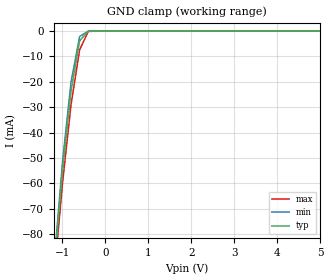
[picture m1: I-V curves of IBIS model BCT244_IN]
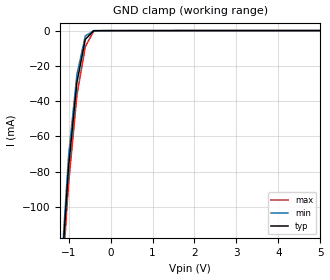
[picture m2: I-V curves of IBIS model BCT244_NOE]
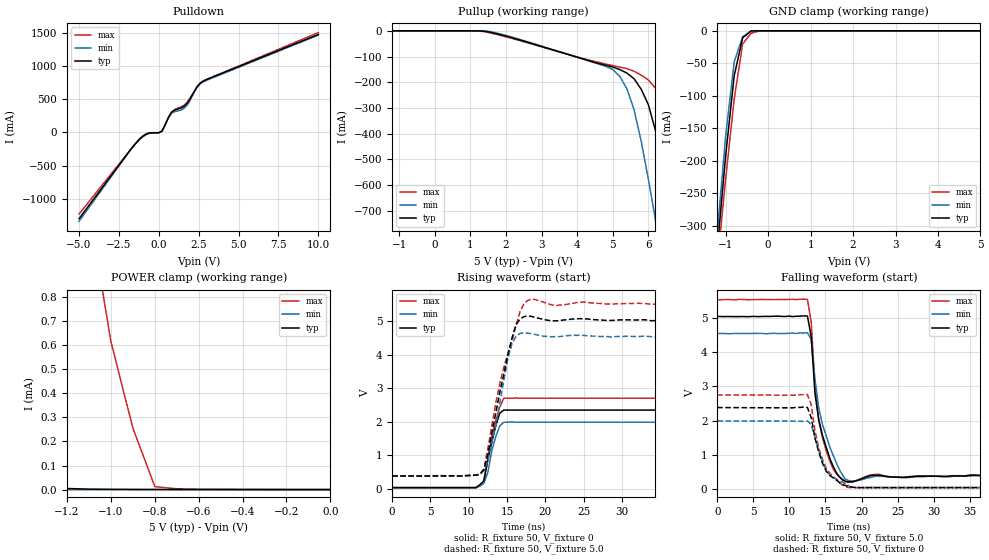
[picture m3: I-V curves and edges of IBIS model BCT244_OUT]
|   TEXAS INSTRUMENTS INCORPORATED
|   Standard Linear and Logic
|   IBIS Model of SN74BCT244
|   OCTAL BUFFERS / DRIVERS WITH 3-STATE OUTPUTS
|   SOIC 20-pin (DW), SOP 20-pin (NS), SSOP 20-pin (DB), PDIP 20-pin (N)
[IBIS Ver]   3.2
[Comment Char]  |_char
[File Name]   sn74bct244.ibs
[File Rev]   4.2 | b_die
[Date]   Oct. 06, 2004
[Source]   File originated at Texas Instruments, Inc.
[Notes]   The following is a sample IBIS file for the BCT244
   - FILE REV HISTORY
   - 4.2 Re-Release IBIS file on 10/08/04
   - All test data contained in this file are derived from
   actual measurements.
   - The measurement used NS package.
   - We have data across voltage and temperature, but not
   across process.
   - As there is no power clamp diode we removed the Pwr Clamp
   table data for IN and NOE.
|   - File created by Nobuhisa Ohtsubo, SLL Product Engineering.
[Disclaimer] Property of Texas Instruments Incorporated.  Unauthorized
   reproduction and/or distribution is strictly prohibited.
   This product is protected under copyright law.
   Created 2000, (C) Copyright 2000, Texas Instruments Inc.,
   All Rights Reserved.
   UNLESS THERE IS A SIGNED, WRITTEN AGREEMENT TO THE
   CONTRARY, TEXAS INSTRUMENTS () IS PROVIDING THE IBIS
   MODELS  AND WITHOUT ANY WARRANTY, EXPRESSED OR
   IMPLIED.  TI assumes no liability for:
   1) the accuracy of the IBIS models provided to your
   company;
   2) the proper functioning of these IBIS Models in your
   design or for any resulting applications; or
   3) infringement of patents, copyrights or intellectual
   property rights resulting from your use of these IBIS
   models.
   TI provides IBIS Models as a service to our customers.
   You and your company shall not distribute, sell or give
   these models to anyone else without prior written
   permission from TI.
   TI reserves the right to make changes to our products or
   to discontinue any semiconductor product or service
   without notice, and advises our customers to obtain the
   latest version of relevant information to verify, before
   placing orders, that the information being relied on is
   current.
   Please be aware that your receipt and use of the IBIS
   information provided shall serve as acceptance of these
   terms and conditions.  If you do not accept these terms,
   you should return or destroy the IBIS models and any
   other accompanying information immediately.
|   Component BCT244_DW
[Component]   BCT244_DW
[Manufacturer]  Texas Instruments, Inc.
[Package]
|   typ   min   max
R_pkg   0.038   0.033   0.045
L_pkg   5.012nH   4.110nH   6.349nH
C_pkg   0.717pF   0.530pF   0.868pF
[Pin]   signal_name   model_name   R_pin   L_pin   C_pin
1   1NOE   BCT244_NOE   0.058   5.115nH   0.725pF
2   1A1   BCT244_IN   0.053   4.591nH   0.724pF
3   2Y4   BCT244_OUT   0.049   3.754nH   0.572pF
4   1A2   BCT244_IN   0.029   2.549nH   0.388pF
5   2Y3   BCT244_OUT   0.031   2.317nH   0.316pF
6   1A3   BCT244_IN   0.031   2.317nH   0.316pF
7   2Y2   BCT244_OUT   0.029   2.556nH   0.399pF
8   1A4   BCT244_IN   0.049   3.754nH   0.579pF
9   2Y1   BCT244_OUT   0.053   4.591nH   0.724pF
10   GND   GND   0.058   5.115nH   0.725pF
11   2A1   BCT244_IN   0.058   5.115nH   0.725pF
12   1Y4   BCT244_OUT   0.053   4.591nH   0.724pF
13   2A2   BCT244_IN   0.049   3.754nH   0.579pF
14   1Y3   BCT244_OUT   0.029   2.557nH   0.399pF
15   2A3   BCT244_IN   0.031   2.317nH   0.316pF
16   1Y2   BCT244_OUT   0.031   2.317nH   0.316pF
17   2A4   BCT244_IN   0.029   2.557nH   0.399pF
18   1Y1   BCT244_OUT   0.049   3.754nH   0.579pF
19   2NOE   BCT244_NOE   0.053   4.591nH   0.724pF
20   VCC   POWER   0.058   5.115nH   0.725pF
|   Component BCT244_NS
[Component]   BCT244_NS
[Manufacturer]  Texas Instruments, Inc.
[Package]
|   typ   min   max
R_pkg   0.044   0.029   0.058
L_pkg   3.666nH   2.317nH   5.115nH
C_pkg   0.548pF   0.316pF   0.725pF
[Pin]   signal_name   model_name   R_pin   L_pin   C_pin
1   1NOE   BCT244_NOE   0.058   5.115nH   0.725pF
2   1A1   BCT244_IN   0.053   4.591nH   0.724pF
3   2Y4   BCT244_OUT   0.049   3.754nH   0.572pF
4   1A2   BCT244_IN   0.029   2.549nH   0.388pF
5   2Y3   BCT244_OUT   0.031   2.317nH   0.316pF
6   1A3   BCT244_IN   0.031   2.317nH   0.316pF
7   2Y2   BCT244_OUT   0.029   2.556nH   0.399pF
8   1A4   BCT244_IN   0.049   3.754nH   0.579pF
9   2Y1   BCT244_OUT   0.053   4.591nH   0.724pF
10   GND   GND   0.058   5.115nH   0.725pF
11   2A1   BCT244_IN   0.058   5.115nH   0.725pF
12   1Y4   BCT244_OUT   0.053   4.591nH   0.724pF
13   2A2   BCT244_IN   0.049   3.754nH   0.579pF
14   1Y3   BCT244_OUT   0.029   2.557nH   0.399pF
15   2A3   BCT244_IN   0.031   2.317nH   0.316pF
16   1Y2   BCT244_OUT   0.031   2.317nH   0.316pF
17   2A4   BCT244_IN   0.029   2.557nH   0.399pF
18   1Y1   BCT244_OUT   0.049   3.754nH   0.579pF
19   2NOE   BCT244_NOE   0.053   4.591nH   0.724pF
20   VCC   POWER   0.058   5.115nH   0.725pF
|   Component BCT244_DB
[Component]   BCT244_DB
[Manufacturer]  Texas Instruments, Inc.
[Package]
|   typ   min   max
R_pkg   0.040   0.035   0.051
L_pkg   3.495nH   3.035nH   4.314nH
C_pkg   0.420pF   0.346pF   0.502pF
[Pin]   signal_name   model_name   R_pin   L_pin   C_pin
1   1NOE   BCT244_NOE   0.049   4.310nH   0.502pF
2   1A1   BCT244_IN   0.048   3.903nH   0.487pF
3   2Y4   BCT244_OUT   0.035   3.189nH   0.396pF
4   1A2   BCT244_IN   0.035   3.036nH   0.347pF
5   2Y3   BCT244_OUT   0.035   3.035nH   0.367pF
6   1A3   BCT244_IN   0.035   3.035nH   0.367pF
7   2Y2   BCT244_OUT   0.035   3.036nH   0.347pF
8   1A4   BCT244_IN   0.035   3.189nH   0.397pF
9   2Y1   BCT244_OUT   0.047   3.899nH   0.488pF
10   GND   GND   0.051   4.314nH   0.500pF
11   2A1   BCT244_IN   0.051   4.314nH   0.500pF
12   1Y4   BCT244_OUT   0.047   3.899nH   0.488pF
13   2A2   BCT244_IN   0.035   3.189nH   0.397pF
14   1Y3   BCT244_OUT   0.035   3.036nH   0.346pF
15   2A3   BCT244_IN   0.035   3.035nH   0.367pF
16   1Y2   BCT244_OUT   0.035   3.035nH   0.367pF
17   2A4   BCT244_IN   0.035   3.036nH   0.346pF
18   1Y1   BCT244_OUT   0.035   3.189nH   0.397pF
19   2NOE   BCT244_NOE   0.047   3.899nH   0.488pF
20   VCC   POWER   0.051   4.314nH   0.502pF
|   Component BCT244_N
[Component]   BCT244_N
[Manufacturer]   Texas Instruments, Inc.
[Package]
|   typ   min   max
R_pkg   4.300e-02   3.800e-02   5.000e-02
L_pkg   7.384e-09   4.680e-09   1.032e-08
C_pkg   5.100e-13   2.310e-13   8.210e-13
[PIN]   signal_name   model_name   R_pin   L_pin   C_pin
1   1NOE   BCT244_NOE   4.200e-02   9.427e-09   8.100e-13
2   1A1   BCT244_IN   4.600e-02   8.544e-09   4.560e-13
3   2Y4   BCT244_OUT   4.800e-02   7.163e-09   4.350e-13
4   1A2   BCT244_IN   4.000e-02   4.825e-09   2.610e-13
5   2Y3   BCT244_OUT   4.000e-02   5.284e-09   6.480e-13
6   1A3   BCT244_IN   4.000e-02   4.686e-09   2.320e-13
7   2Y2   BCT244_OUT   4.000e-02   6.359e-09   4.890e-13
8   1A4   BCT244_IN   3.800e-02   7.982e-09   4.750e-13
9   2Y1   BCT244_OUT   4.300e-02   9.403e-09   4.750e-13
10   GND   GND   5.000e-02   1.032e-08   8.050e-13
11   2A1   BCT244_IN   5.000e-02   1.028e-08   8.100e-13
12   1Y4   BCT244_OUT   4.300e-02   9.383e-09   4.770e-13
13   2A2   BCT244_IN   3.800e-02   7.978e-09   4.760e-13
14   1Y3   BCT244_OUT   4.000e-02   6.302e-09   4.920e-13
15   2A3   BCT244_IN   4.000e-02   4.680e-09   2.310e-13
16   1Y2   BCT244_OUT   4.000e-02   5.284e-09   6.480e-13
17   2A4   BCT244_IN   4.000e-02   4.822e-09   2.610e-13
18   1Y1   BCT244_OUT   4.700e-02   7.118e-09   4.390e-13
19   2NOE   BCT244_NOE   4.600e-02   8.492e-09   4.610e-13
20   VCC   POWER   4.300e-02   9.348e-09   8.210e-13
| Models and submodels in the file (3): BCT244_IN (Input), BCT244_NOE (Input), BCT244_OUT (3-state)
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|   Model BCT244_IN
[Model]   BCT244_IN
Model_type  Input
Polarity   Inverting
Vinl = 0.8
Vinh = 2.0
| variable   typ   min   max
C_comp   1.33pf   1.00pf   1.66pf
[Temperature Range]   25   0   70
[Voltage Range]   5.0   4.5   5.5
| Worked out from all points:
|   GND clamp passes 1 mA (typ) near -0.45 V on its own axis
[GND Clamp]
|   Voltage   I(typ)   I(min)   I(max)
-5V       -1.129A    -1.189A    -1.042A
-1.2V     -95.01mA   -92.75mA   -98.11mA
-1V       -55.16mA   -51.8mA    -60.26mA
-800mV    -23.57mA   -20.06mA   -29.07mA
-600mV    -3.849mA   -2.148mA   -7.399mA
-400mV    -30.54uA   -20.12uA   -154.2uA
5V        3.151nA    4.209nA    5.215nA
|   Model BCT244_NOE
[Model]   BCT244_NOE
Model_type  Input
Polarity   Inverting
Vinl = 0.8
Vinh = 2.0
| variable   typ   min   max
C_comp   1.33pf   1.00pf   1.66pf
[Temperature Range]   25   0   70
[Voltage Range]   5.0   4.5   5.5
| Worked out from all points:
|   GND clamp passes 1 mA (typ) near -0.44 V on its own axis
[GND Clamp]
|   Voltage   I(typ)   I(min)   I(max)
-5V       -1.905A    -1.987A    -1.775A
-1.2V     -149.5mA   -144.7mA   -156.5mA
-1V       -77.36mA   -71.2mA    -87.15mA
-800mV    -29.14mA   -24.72mA   -36.51mA
-600mV    -4.94mA    -2.996mA   -9.102mA
-400mV    -73.28uA   -48.98uA   -291.7uA
5V        3.575nA    6.334nA    4.663nA
|   Model BCT244_OUT
[Model]   BCT244_OUT
Model_type  3-state
Polarity   Non-Inverting
Vmeas = 1.3v
Cref = 50pF
Rref = 500
Vref = 0
| variable   typ   min   max
C_comp   5.8pf   4.35pf   7.25pf
[Temperature Range]   25   0   70
[Voltage Range]   5.0   4.5   5.5
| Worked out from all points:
|   slope of the pulldown table from 0 to 0.75 V, typ, clamps not added: 2.58 ohm
|   slope of the pullup table from 0 to 0.75 V, typ, clamps not added: 69.6 kohm
|   GND clamp passes 1 mA (typ) near -0.41 V on its own axis
|   POWER clamp passes 1 mA (typ) near -1.49 V on its own axis
|   rising waveform, R_fixture 50, V_fixture 0: 20-80 % time 1.33ns typ, 1.2ns min, 1.48ns max; typ from 0.031 V to 2.35 V
|   falling waveform, R_fixture 50, V_fixture 5.0: 20-80 % time 1.83ns typ, 2.31ns min, 1.56ns max; typ from 5.05 V to 0.385 V
|   rising waveform, R_fixture 50, V_fixture 5.0: 20-80 % time 2.5ns typ, 2.1ns min, 3.1ns max; typ from 0.375 V to 5.05 V
|   falling waveform, R_fixture 50, V_fixture 0: 20-80 % time 1.97ns typ, 2.1ns min, 1.95ns max; typ from 2.38 V to 0.038 V
[Pulldown]
|   Voltage   I(typ)   I(min)   I(max)
-5V       -1.301A    -1.34A     -1.231A
-1.4V     -150mA     -146.8mA   -155.5mA
-800mV    -25.67mA   -22.18mA   -32.16mA
0V        -3.555mA   -3.081mA   -3.835mA
200mV     20.62mA    17.38mA    24.14mA
600mV     226.1mA    225.5mA    220.1mA
800mV     306.8mA    292.7mA    307mA
1.4V      369.7mA    339.2mA    386mA
1.8V      446.6mA    417.2mA    464.2mA
2.4V      689.8mA    684.3mA    687.6mA
2.6V      747mA      735.8mA    746.7mA
10V       1.48A      1.47A      1.508A
[Pullup]
|   Voltage   II(typ)   I(min)   I(max)
-5V       358.5nA    32.07nA    1.938uA
1.6V      -6.726mA   -3.915mA   -9.483mA
4.8V      -133.8mA   -138.1mA   -129mA
5.4V      -164.5mA   -225.5mA   -147mA
5.8V      -226.9mA   -428.3mA   -172.3mA
6.2V      -386.1mA   -732.6mA   -222.7mA
6.4V      -515mA     -890.3mA   -269.8mA
6.6V      -658.1mA   -1.048A    -350.3mA
6.8V      -804.3mA   -1.206A    -460.9mA
7.2V      -1.097A    -1.521A    -723.4mA
7.4V      -1.243A    -1.679A    -858.6mA
10V       -3.144A    -3.729A    -2.616A
[GND Clamp]
|   Voltage   I(typ)   I(min)   I(max)
-5V       -3.404A    -3.589A    -3.148A
-1.2V     -336.9mA   -312.6mA   -359.9mA
-1V       -192mA     -161.5mA   -227.6mA
-800mV    -69.25mA   -47.96mA   -105.1mA
-600mV    -10.72mA   -9.275mA   -20.06mA
-400mV    -238.4uA   -59.33uA   -3.69mA
-200mV    -406.9nA   -35.2nA    -6.329uA
5V        7.479nA    7.498nA    11.84nA
[POWER Clamp]
|   Voltage   I(typ)   I(min)   I(max)
-5V       18.8mA     15.37mA    21.39mA
-1.9V     3.29mA     895.8uA    5.406mA
-1.8V     2.763mA    395.4uA    4.891mA
-1.7V     2.21mA     90.41uA    4.375mA
-1.5V     1.037mA    1.268uA    3.344mA
-1.3V     161uA      495.3nA    2.292mA
-1.2V     4.54uA     339.7nA    1.736mA
-1.1V     1.955uA    240.5nA    1.165mA
-1V       1.128uA    174.3nA    613.8uA
-900mV    725.4nA    129.1nA    255.1uA
-800mV    492.1nA    96.78nA    12.22uA
0V        47.33nA    16.28nA    223.5nA
[Ramp]
| variable   typ   min   max
dV/dt_r  1.344E+00/1.196E-09  1.110E+00/1.113E-09  1.584E+00/1.402E-09
dV/dt_f  2.874E+00/1.782E-09  2.568E+00/2.198E-09  3.174E+00/1.484E-09
R_load = 50
[Rising Waveform]
R_fixture = 50
V_fixture = 0
V_fixture_min = 0
V_fixture_max = 0
C_fixture = 0pf
L_fixture = 0nH
|   Time   V(typ)   V(min)   V(max)
0s        30.99mV    20.28mV    21.99mV
10.94ns   30.97mV    20.22mV    21.01mV
11.46ns   115.4mV    71.96mV    81.93mV
11.98ns   222.6mV    155mV      254.5mV
12.5ns    848.1mV    477.3mV    895.9mV
13.02ns   1.404V     1.136V     1.567V
13.54ns   1.884V     1.556V     2.031V
14.06ns   2.255V     1.874V     2.444V
14.58ns   2.349V     1.983V     2.699V
50ns      2.347V     1.984V     2.7V
[Falling Waveform]
R_fixture = 50
V_fixture = 5.0
V_fixture_min = 4.5
V_fixture_max = 5.5
C_fixture = 0pf
L_fixture = 0nH
|   Time   V(typ)   V(min)   V(max)
0s        5.05V      4.552V     5.537V
12.5ns    5.062V     4.573V     5.549V
13.02ns   4.457V     4.379V     4.892V
13.54ns   2.803V     3.219V     3.037V
14.06ns   2.027V     2.378V     2.012V
15.63ns   875.7mV    1.208V     791.5mV
16.67ns   418.7mV    681.6mV    400.5mV
17.71ns   226.4mV    289.9mV    211.6mV
22.4ns    403.9mV    371.3mV    428.6mV
50ns      385mV      375.1mV    389.3mV
[Rising Waveform]
R_fixture = 50
V_fixture = 5.0
V_fixture_min = 4.5
V_fixture_max = 5.5
C_fixture = 0pf
L_fixture = 0nH
|   Time   V(typ)   V(min)   V(max)
0s        375.1mV    377.7mV    385.1mV
10.94ns   398.1mV    403.1mV    402.7mV
11.98ns   568.9mV    526.3mV    575.7mV
12.5ns    1.017V     840mV      1.2V
14.06ns   2.882V     2.56V      3.145V
15.1ns    3.986V     3.868V     4.028V
15.63ns   4.486V     4.317V     4.39V
16.67ns   5.062V     4.64V      5.276V
17.71ns   5.165V     4.649V     5.629V
50ns      5.047V     4.55V      5.541V
[Falling Waveform]
R_fixture = 50
V_fixture = 0
V_fixture_min = 0
V_fixture_max = 0
C_fixture = 0pf
L_fixture = 0nH
|   Time   V(typ)   V(min)   V(max)
0s        2.382V     1.989V     2.747V
12.5ns    2.383V     1.988V     2.763V
13.02ns   2.087V     1.879V     2.468V
13.54ns   1.498V     1.516V     1.708V
14.06ns   1.083V     1.141V     1.2V
14.58ns   753mV      804mV      867.5mV
15.63ns   389.7mV    391.7mV    448.2mV
17.71ns   99.79mV    160.7mV    64.24mV
18.75ns   50.5mV     30.48mV    44.4mV
50ns      38.24mV    32.21mV    43.38mV
